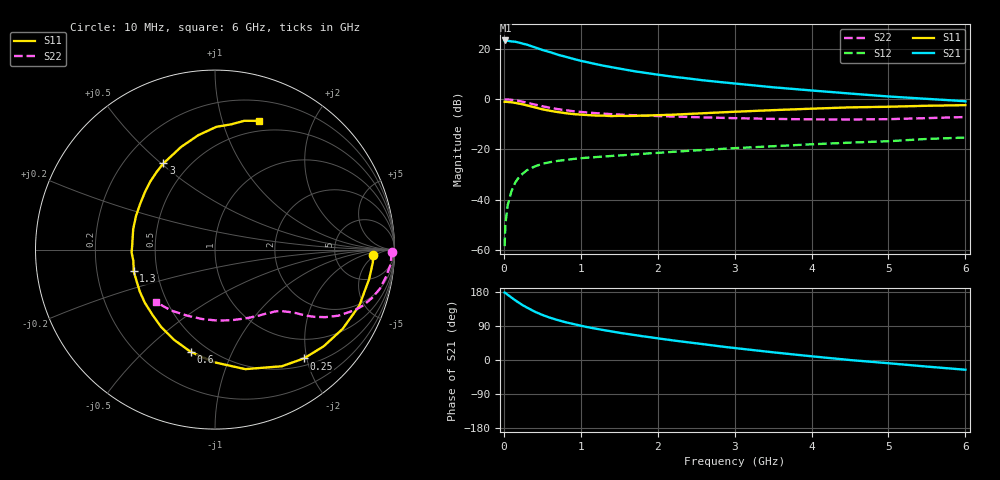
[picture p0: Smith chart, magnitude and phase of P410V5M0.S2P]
! SIEMENS Small Signal Semiconductors
! BFP182
! Si NPN RF Bipolar Junction Transistor in SOT143
! VCE = 10 V  IC = 5 mA
! Common Emitter S-Parameters:  March  1996
# GHz  S  MA  R  50
!  f  S11  S21  S12  S22
! GHz  MAG  ANG  MAG  ANG  MAG  ANG  MAG  ANG
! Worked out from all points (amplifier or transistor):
!   36 points, 10 MHz to 6 GHz, reference 50 ohm
!   highest |S21| = 23.3 dB at 20 MHz (marker M1)
!   |S21| within 3 dB of that: start of sweep to 428.5 MHz
!   unconditionally stable (mu >= 1): 1.675 GHz to 5.894 GHz
!   at 250 MHz: K = 0.21, MSG = 25.7 dB, |S12| = -29.5 dB
!   at 1.4 GHz: K = 0.90, MSG = 17.6 dB, |S12| = -22.6 dB
!   at 6 GHz: K = 0.99, MSG = 7.2 dB, |S12| = -15.3 dB
!   S11 on the Smith chart (normalised r, x): 10 MHz: 15, -4; 250 MHz: 0.62, -1.95; 600 MHz: 0.41, -0.71; 1.3 GHz: 0.37, -0.11; 3 GHz: 0.36, +0.51; 6 GHz: 0.39, +1.32
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0.01  0.8808 -2.1  14.4 178.0  0.0012 81.0  0.9884 -0.9
0.02  0.8823 -4.6  14.58 177.0  0.0033 85.5  0.9829 -1.8
0.05  0.8744 -10.8  14.36 172.2  0.0078 87.3  0.9828 -4.6
0.15  0.8369 -31.9  13.73 157.3  0.0222 72.0  0.9439 -13.4
0.2  0.8104 -41.7  13.18 150.5  0.0286 67.7  0.9156 -17.1
0.25  0.7827 -50.8  12.54 144.0  0.0335 63.2  0.883 -20.6
0.3  0.749 -60.2  12.03 138.5  0.0386 59.3  0.8463 -23.6
0.4  0.687 -75.8  10.69 127.7  0.0458 52.6  0.7795 -28.2
0.5  0.6272 -90.6  9.459 119.0  0.052 47.3  0.7221 -31.4
0.6  0.5858 -103.3  8.547 111.6  0.0558 43.7  0.6723 -33.9
0.7  0.552 -114.4  7.609 105.4  0.0593 41.3  0.6318 -35.7
0.8  0.5251 -124.9  6.936 99.8  0.0618 38.9  0.6005 -37.0
1  0.4905 -142.8  5.748 90.5  0.0669 35.9  0.5555 -39.1
1.1  0.4799 -150.8  5.33 86.2  0.0689 35.3  0.5379 -40.2
1.3  0.4688 -165.0  4.585 78.9  0.0723 33.9  0.5119 -42.1
1.7  0.4638 171.3  3.564 65.9  0.0798 33.0  0.4769 -46.5
2.2  0.489 148.4  2.779 51.7  0.0896 32.0  0.4504 -53.2
3  0.5598 120.9  2.038 31.6  0.1061 29.3  0.4176 -66.9
3.5  0.6026 108.2  1.714 20.3  0.1157 27.1  0.4039 -77.1
4.5  0.6839 89.4  1.288 -0.1  0.1363 22.1  0.3933 -100.6
5.5  0.736 77.2  1.01 -17.4  0.1615 17.4  0.4183 -125.8
6  0.7571 71.3  0.905 -25.7  0.1722 13.5  0.4398 -138.2
